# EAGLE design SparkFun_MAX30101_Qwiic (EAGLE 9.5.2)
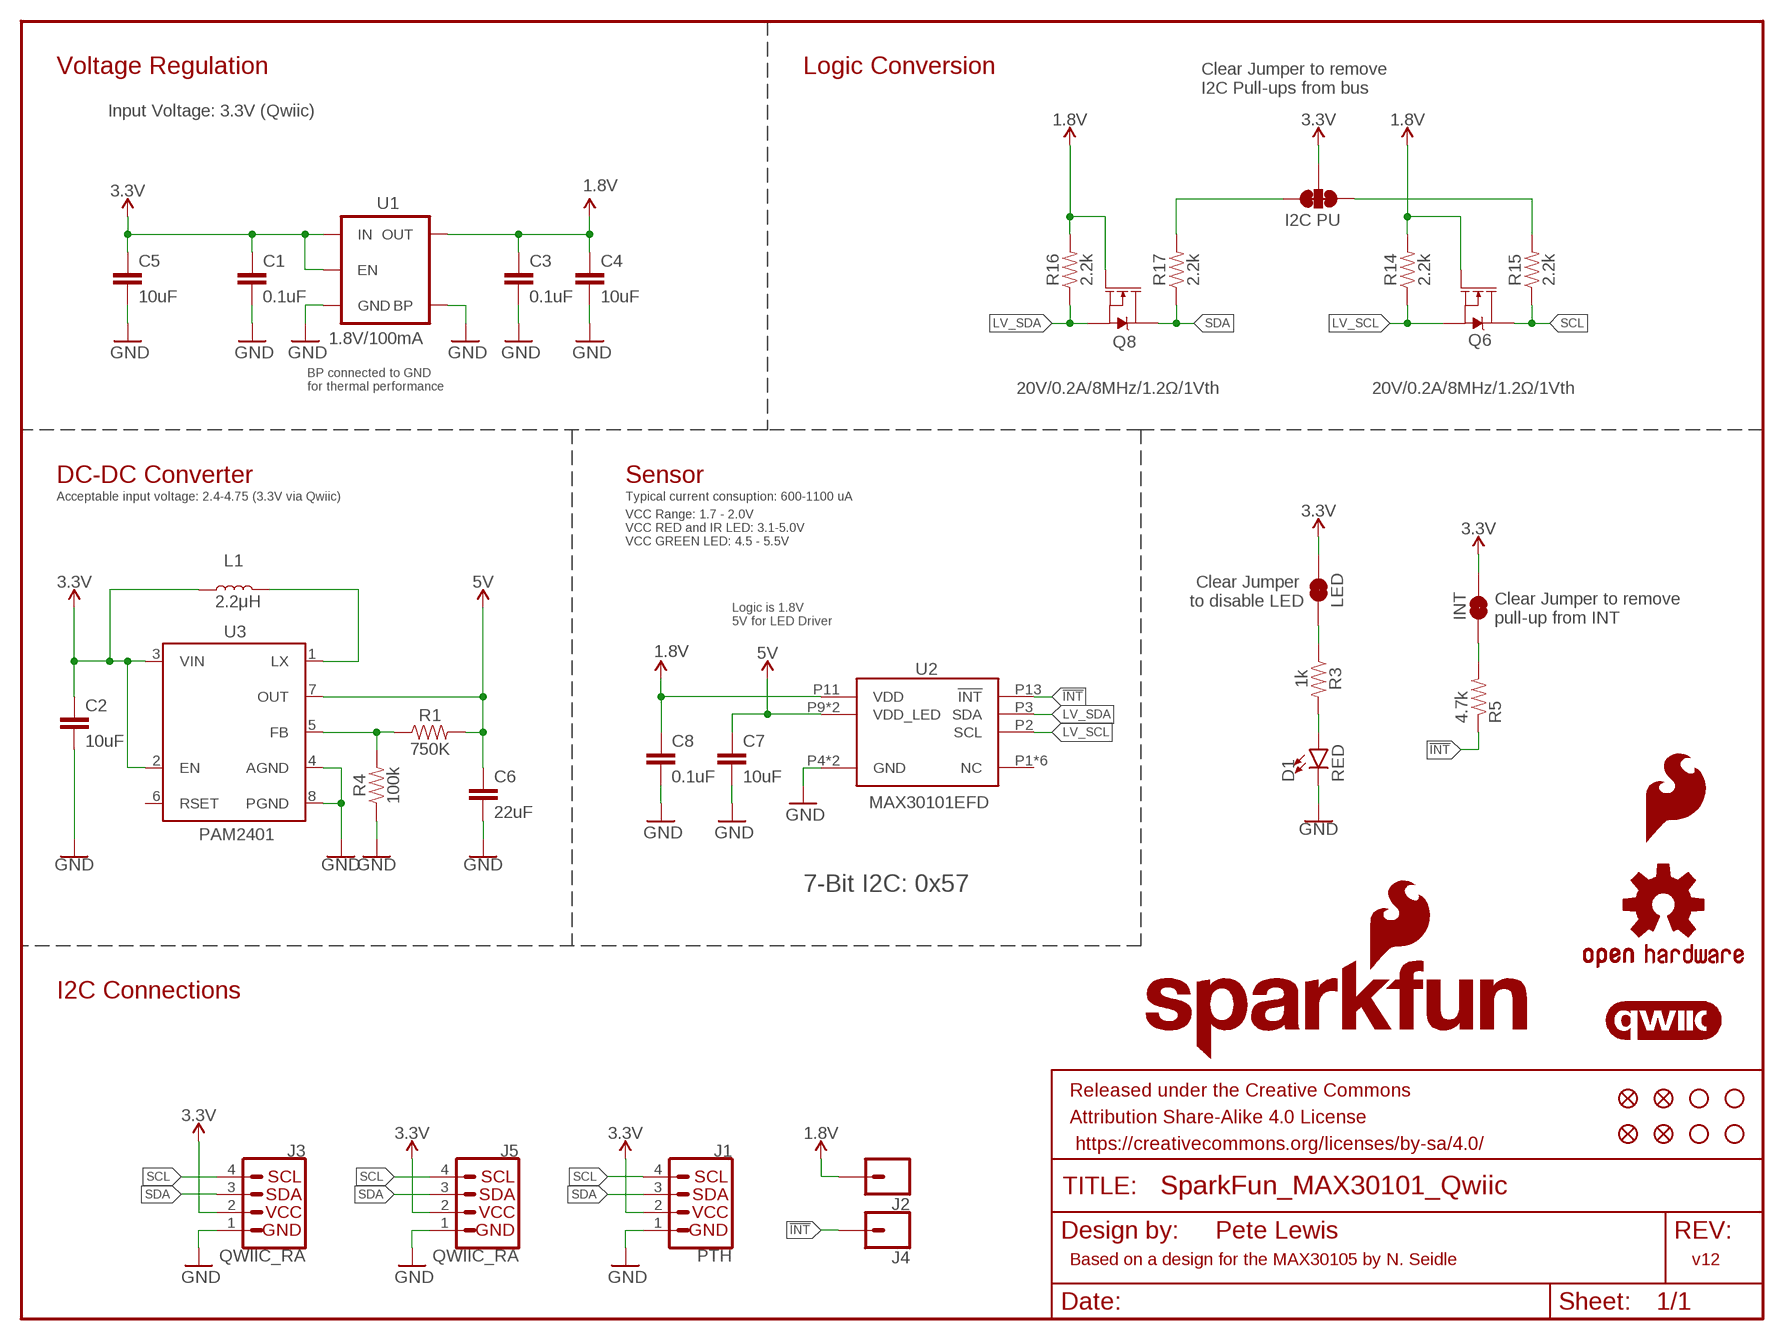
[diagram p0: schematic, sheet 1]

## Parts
C1  0.1uF  0.1UF-0402-16V-10%  [0402]
C2  10uF  10UF-0603-6.3V-20%  [0603]
C3  0.1uF  0.1UF-0402-16V-10%  [0402]
C4  10uF  10UF-0603-6.3V-20%  [0603]
C5  10uF  10UF-0603-6.3V-20%  [0603]
C6  22uF  22UF-0805-6.3V-20%  [0805]
C7  10uF  10UF-0603-6.3V-20%  [0603]
C8  0.1uF  0.1UF-0402-16V-10%  [0402]
D1  RED  LED-RED0603  [LED-0603]
FID1  FIDUCIAL1X2  [FIDUCIAL-1X2]
FID2  FIDUCIAL1X2  [FIDUCIAL-1X2]
FID3  FIDUCIAL1X2  [FIDUCIAL-1X2]
FID4  FIDUCIAL1X2  [FIDUCIAL-1X2]
FRAME1  FRAME-LETTER  [CREATIVE_COMMONS]
J1  PTH  I2C_STANDARD_NO_SILK  [1X04_NO_SILK]
J2  CONN_01PTH_NO_SILK_YES_STOP  [1X01_NO_SILK]
J3  QWIIC_RA  QWIIC_CONNECTORJS-1MM  [JST04_1MM_RA]
J4  CONN_01PTH_NO_SILK_YES_STOP  [1X01_NO_SILK]
J5  QWIIC_RA  QWIIC_CONNECTORJS-1MM  [JST04_1MM_RA]
JP1  LED  JUMPER-SMT_2_NC_TRACE_SILK  [SMT-JUMPER_2_NC_TRACE_SILK]
JP2  INT  JUMPER-SMT_2_NC_TRACE_SILK  [SMT-JUMPER_2_NC_TRACE_SILK]
JP4  I2C PU  JUMPER-SMT_3_2-NC_TRACE_SILK  [SMT-JUMPER_3_2-NC_TRACE_SILK]
L1  2.2μH  2.2μH_SHIELDED_INDUCTOR  [0806]
LOGO1  SFE_LOGO_NAME_FLAME.1_INCH  [SFE_LOGO_NAME_FLAME_.1]
LOGO2  OSHW-LOGOS  [OSHW-LOGO-S]
LOGO3  QWIIC_LOGO_5MM  [QWIIC_5MM]
LOGO4  SFE_LOGO_FLAME.1_INCH  [SFE_LOGO_FLAME_.1]
Q6  20V/0.2A/8MHz/1.2Ω/1Vth  MOSFET-NCH-RE1C00UNTL  [SOT-416FL]
Q8  20V/0.2A/8MHz/1.2Ω/1Vth  MOSFET-NCH-RE1C00UNTL  [SOT-416FL]
R1  750K  750KOHM-0603-1/10W-1%  [0603]
R3  1k  1KOHM-0603-1/10W-1%  [0603]
R4  100k  100KOHM-0603-1/10W-1%  [0603]
R5  4.7k  4.7KOHM-0603-1/10W-1%  [0603]
R14  2.2k  2.2KOHM-0603-1/10W-1%  [0603]
R15  2.2k  2.2KOHM-0603-1/10W-1%  [0603]
R16  2.2k  2.2KOHM-0603-1/10W-1%  [0603]
R17  2.2k  2.2KOHM-0603-1/10W-1%  [0603]
STANDOFF1  STAND-OFF  [STAND-OFF]
STANDOFF2  STAND-OFF  [STAND-OFF]
STANDOFF3  STAND-OFF  [STAND-OFF]
STANDOFF4  STAND-OFF  [STAND-OFF]
U1  1.8V/100mA  V_REG_SP62141.8V  [SC70]
U2  MAX30101EFD  [14_PIN_OESIP]
U3  PAM2401  [MSOP8]

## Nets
1.8V: C3.1 C4.1 C8.1 J2.1 Q6.1(G) Q8.1(G) R14.2 R16.2 U1.5(OUT) U2.P11(VDD)
3.3V: C1.1 C2.1 C5.1 J1.2 J3.2 J5.2 JP1.2 JP2.2 JP4.2 L1.1 U1.1(IN) U1.3(EN) U3.2(EN) U3.3(VIN)
5V: C6.1 C7.1 R1.2 U2.P9(VDD_LED) U2.P10(VDD_LED) U3.7(OUT)
!INT: J4.1 R5.1 U2.P13(!INT)
GND [power]: C1.2 C2.2 C3.2 C4.2 C5.2 C6.2 C7.2 C8.2 D1.C J1.1 J3.1 J5.1 R4.1 U1.2(GND) U1.4(BP) U2.P4(GND) U2.P12(GND) U3.4(AGND) U3.8(PGND)
LV_SCL: Q6.2(S) R14.1 U2.P2(SCL)
LV_SDA: Q8.2(S) R16.1 U2.P3(SDA)
N$1: JP2.1 R5.2
N$2: R1.1 R4.2 U3.5(FB)
N$3: L1.2 U3.1(LX)
N$4: D1.A R3.2
N$5: JP4.3 R15.2
N$6: JP4.1 R17.2
N$8: JP1.1 R3.1
SCL: J1.4 J3.4 J5.4 Q6.3(D) R15.1
SDA: J1.3 J3.3 J5.3 Q8.3(D) R17.1
Unconnected: U2.P1(NC) U2.P5(NC) U2.P6(NC) U2.P7(NC) U2.P8(NC) U2.P14(NC) U3.6(RSET)

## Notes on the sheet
- Voltage Regulation | Logic Conversion
- Clear Jumper to remove 
  I2C Pull-ups from bus
- Input Voltage: 3.3V (Qwiic)
- BP connected to GND
  for thermal performance
- DC-DC Converter | Sensor
- Acceptable input voltage: 2.4-4.75 (3.3V via Qwiic) | Typical current consuption: 600-1100 uA
- VCC Range: 1.7 - 2.0V
  VCC RED and IR LED: 3.1-5.0V
  VCC GREEN LED: 4.5 - 5.5V
- Clear Jumper 
  to disable LED
- Clear Jumper to remove 
  pull-up from INT
- Logic is 1.8V
  5V for LED Driver
- 7-Bit I2C: 0x57
- I2C Connections
- Pete Lewis
- Based on a design for the MAX30105 by N. Seidle | v12

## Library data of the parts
C1 C3 C8 = SparkFun-Capacitors:0.1UF: 0.1µF ceramic capacitors; PROD_ID: CAP-12416
C2 C4 C5 C7 = SparkFun-Capacitors:10UF: 10.0µF ceramic capacitors; PROD_ID: CAP-11015
C6 = SparkFun-Capacitors:22UF: 22µF ceramic capacitors; PROD_ID: CAP-08402
D1 = SparkFun-LED:LED-RED: Red SMD LED; PROD_ID: DIO-00819
FID1-FID4 = SparkFun-Aesthetics:FIDUCIAL: Fiducial Alignment Points
FRAME1 = SparkFun-Aesthetics:FRAME-LETTER: Schematic Frame - Letter
J1 = SparkFun-Connectors:I2C_STANDARD: SparkFun I2C Standard Pinout Header SparkFun has standardized on a pinout for all I2C based sensor breakouts. This pinout allows I2C boards to be plugged directly into the headers on Arduino Uno compatible boards, and to be daisy chained easily. Example SparkFun Products: SparkFun Atmospheric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
J2 J4 = SparkFun-Connectors:CONN_01: Single connection point. Often used as Generic Header-pin footprint for 0.1 inch spaced/style header connections
J3 J5 = SparkFun-Connectors:QWIIC_CONNECTOR: SparkFun I2C Standard Qwiic Connector An SMD 1mm pitch JST connector makes it easy and quick (get it? Qwiic?) to connect I2C devices to each other. The Qwiic system enables fast and solderless connection between popular platforms and various sensors and actuators. We carry 200mm, 100mm, 50mm, and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; PROD_ID: CONN-13694; VALUE: QWIIC_RIGHT_ANGLE
JP1 JP2 = SparkFun-Jumpers:JUMPER-SMT_2_NC_TRACE: Normally closed trace jumper
JP4 = SparkFun-Jumpers:JUMPER-SMT_3_2-NC_TRACE: Normally closed trace jumper (2 of 2 connections) This jumper has a trace between all three pads so they are normally closed (NC). Use a razor knife to open the connection(s). For best results follow the IPC guidelines for cutting traces: Cutout at least 0.063 mm (0.005 in). Remove all loose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
L1 = SparkFun-Coils:2.2μH_SHIELDED_INDUCTOR: Murata 2.2uH Inductor; PROD_ID: NDUC-14257
LOGO1 = SparkFun-Aesthetics:SFE_LOGO_NAME_FLAME: SparkFun Font Logo w/ Flame
LOGO2 = SparkFun-Aesthetics:OSHW-LOGO: Open-Source Hardware (OSHW) Logo
LOGO3 = SparkFun-Aesthetics:QWIIC_LOGO: Qwiic Logos for placement on schematic and PCB. The 5.5mm silk logo is best for placing next to Qwiic connector.
LOGO4 = SparkFun-Aesthetics:SFE_LOGO_FLAME: SparkFun Flame Logo
Q6 Q8 = SparkFun-DiscreteSemi:MOSFET-NCH: N-channel MOSFETs Voltage controlled devices that allow control of high current outputs. SparkFun Products: SparkFun OpenScale SparkFun Digital Sandbox SparkFun Monster Moto Shield SparkFun MOSFET Power Controller; PROD_ID: TRANS-14399
R1 = SparkFun-Resistors:750KOHM: 750Ω resistor; PROD_ID: RES-13768
R3 = SparkFun-Resistors:1KOHM: 1kΩ resistor; PROD_ID: RES-07856
R4 = SparkFun-Resistors:100KOHM: 100kΩ resistor; PROD_ID: RES-07828
R5 = SparkFun-Resistors:4.7KOHM: 4.7kΩ resistor; PROD_ID: RES-07857
R14-R17 = SparkFun-Resistors:2.2KOHM: 2.2kΩ resistor; PROD_ID: RES-08272
STANDOFF1-STANDOFF4 = SparkFun-Electromechanical:STAND-OFF: #4 Stand Off
U1 = SparkFun-PowerIC:V_REG_SP6214; PROD_ID: VREG-08428
U2 = SparkFun-IC-Special-Function:MAX30101EFD: MAX30101 High-Sensitivity Pulse Oximeter and Heart-Rate Sensor The MAX30101 is an integrated pulse oximetry and heart-rate monitor module. It includes internal LEDs, photodetectors, optical elements, and low-noise electronics with ambient light rejection. The MAX30101 provides a complete system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; PROD_ID: IC-14270
U3 = SparkFun-IC-Power:PAM2401: PAM2401 - Boost PMIC Specifications: Up to 1A output current 0.9V to 4.75V Input Range 2.5V to 5.0V Adjustable Output Voltage Datasheet (Diodes inc.); PROD_ID: IC-13769

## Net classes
1 power: width 0.203 mm

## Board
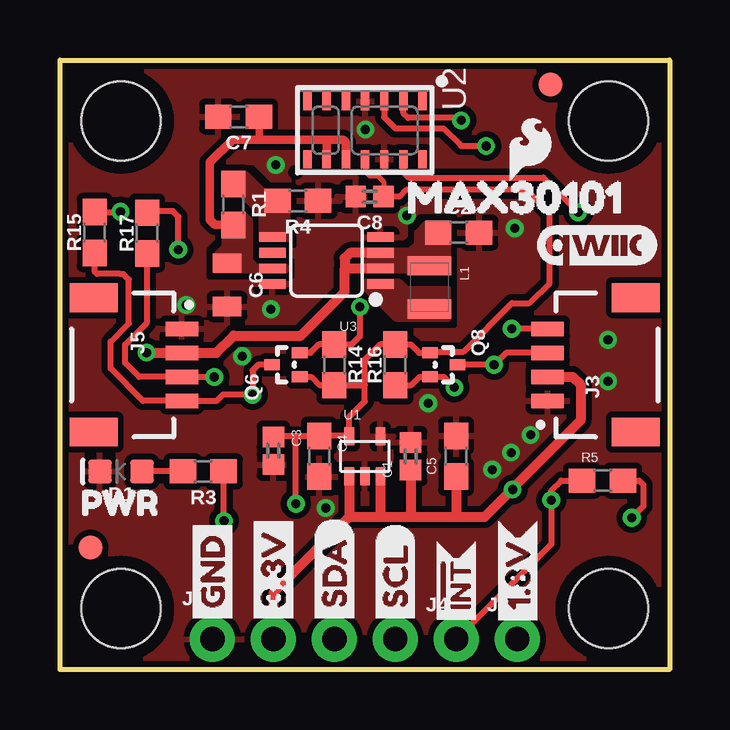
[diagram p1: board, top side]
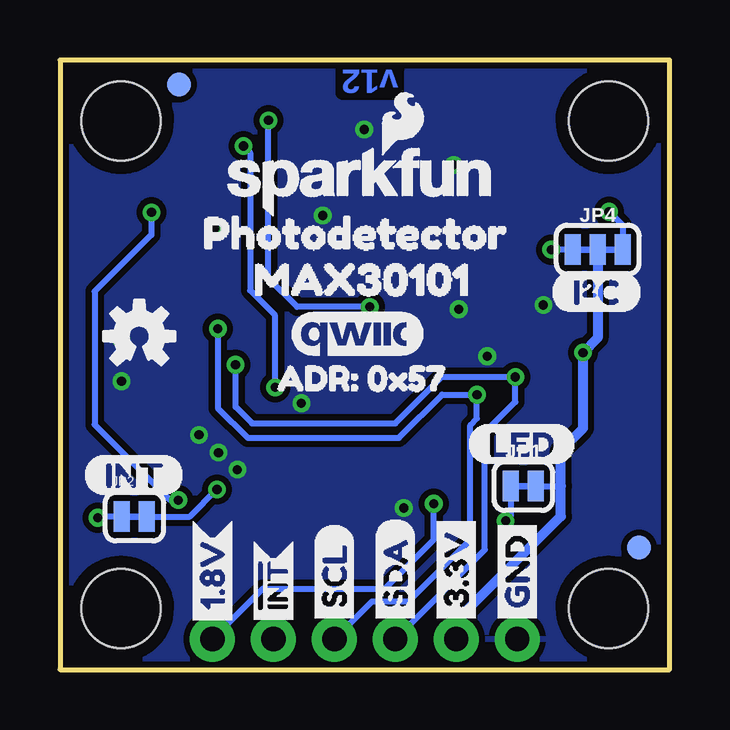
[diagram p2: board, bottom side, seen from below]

Size 25.4 x 25.4 mm. Coordinates in mm from the lower left corner, seen from the top.
Outline: 25.4,25.4 25.4,0 0,0 0,25.4 25.4,25.4
Copper layers (1*16): Top 0.035mm / dielectric 1.5mm / Bottom 0.035mm
Design rules "SparkFun-2-layer-TIGHT": minimum track width 7mil, minimum drill 15mil, track to track 7mil, track to pad 7mil, pad to pad 7mil, via to via 7mil, smd to smd 7mil, copper to edge 7mil, drill to drill 7mil, minimum pad ring 7mil, minimum via ring 7mil, stop-mask expansion 4mil, vias tented up to drill 25mil, thermal gap 10mil

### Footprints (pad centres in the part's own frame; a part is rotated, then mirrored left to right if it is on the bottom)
0402 = smd 0.85 x 0.9: 1 -0.58,0; 2 0.58,0
0603 = smd 1.1 x 1: 1 -0.85,0; 2 0.85,0
0805 = smd 0.8 x 1.2: 1 -0.9,0; 2 0.9,0
LED-0603 = smd 1 x 1: A -0.877,0; C 0.877,0
FIDUCIAL-1X2 = smd 1 x 1: 1 0,0
1X04_NO_SILK = drill 1.016 pad 1.88: 1 0,0; 2 2.54,0; 3 5.08,0; 4 7.62,0
1X01_NO_SILK = drill 1.016 pad 1.88: 1 0,0
JST04_1MM_RA = smd 0.6 x 1.35: 1 -1.5,0; 2 -0.5,0; 3 0.5,0; 4 1.5,0 | smd 1.2 x 2: NC1 2.8,-3.675; NC2 -2.8,-3.675
SMT-JUMPER_2_NC_TRACE_SILK = smd 0.66 x 1.27: 1 -0.521,0; 2 0.521,0
SMT-JUMPER_3_2-NC_TRACE_SILK = smd 0.66 x 1.27: 1 -1.041,0; 2 0,0; 3 1.041,0
0806 = smd 0.8 x 1.8: 1 -0.9,0; 2 0.9,0
SOT-416FL = smd 0.46 x 0.65: 1 -0.5,-1.1; 2 0.5,-1.1; 3 0,0.05
STAND-OFF = hole 3.302: 0,0
SC70 = smd 0.4 x 0.75: 1 -0.65,-0.825; 2 0,-0.825; 3 0.65,-0.825; 4 0.65,0.825; 5 -0.65,0.825
14_PIN_OESIP = smd 0.75 x 0.35: P1 -1.193,2.409; P2 -1.193,1.609; P3 -1.193,0.809; P4 -1.193,0.009; P5 -1.193,-0.791; P6 -1.193,-1.591; P7 -1.193,-2.391; P8 1.207,-2.391; P9 1.207,-1.591; P10 1.207,-0.791; P11 1.207,0.009; P12 1.207,0.809; P13 1.207,1.609; P14 1.207,2.409
MSOP8 = smd 0.4 x 1.1: 1 -0.975,-2.25; 2 -0.325,-2.25; 3 0.325,-2.25; 4 0.975,-2.25; 5 0.975,2.25; 6 0.325,2.25; 7 -0.325,2.25; 8 -0.975,2.25

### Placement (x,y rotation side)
C1  14.61,8.89 90 top
C2  16.61,18.21 0 top
C3  8.89,9.12 270 top
C4  10.79,8.89 270 top
C5  16.51,8.89 90 top
C6  6.96,16.03 270 top
C7  7.44,23.04 180 top
C8  12.9,19.71 180 top
D1  2.54,8.26 180 top
FID1  20.45,24.38 90 top
FID2  1.27,5.08 90 top
FID3  20.45,24.38 0 bottom
FID4  1.27,5.08 0 bottom
FRAME1  not placed on the board
J1  6.35,1.27 0 top
J2  19.05,1.27 0 top
J3  20.32,12.7 90 top
J4  16.51,1.27 0 top
J5  5.08,12.7 270 top
JP1  6.1,7.65 0 bottom
JP2  22.3,6.38 0 bottom
JP4  3,17.5 0 bottom
L1  15.39,15.93 270 top
LOGO1  12.85,20.35 0 bottom
LOGO2  22.1,13.89 0 bottom
LOGO3  22.35,17.7 0 top
LOGO4  19.58,21.69 0 top
Q6  8.89,12.7 90 top
Q8  16.51,12.7 270 top
R1  7.21,19.38 270 top
R3  5.97,8.26 180 top
R4  9.91,19.53 180 top
R5  22.61,7.87 0 top
R14  11.43,12.7 270 top
R15  1.45,18.21 90 top
R16  13.97,12.7 90 top
R17  3.63,18.19 90 top
STANDOFF1  2.54,22.86 90 top
STANDOFF2  22.86,22.86 90 top
STANDOFF3  22.86,2.54 90 top
STANDOFF4  2.54,2.54 90 top
U1  12.7,8.89 0 top
U2  12.7,22.48 270 top
U3  11.1,17.04 90 top
U$1  [PHOTODETECTOR3]  20.6,18.19 0 bottom
U$3  [INT#-[<-04]  16.51,1.4 90 top
U$4  [MAX301010]  13.31,19.68 0 top
U$7  [INT-()-04]  24.46,8.1 0 bottom
U$8  [LED0]  8.46,9.4 0 bottom
U$9  [SCL-[)]  13.97,1.65 90 bottom
U$10  [GND-04]  6.35,1.65 90 top
U$11  [INT#-[<-04]  16.51,1.4 90 bottom
U$12  [SCL-[)]  13.97,1.65 90 top
U$13  [SDA-[)]  11.43,1.65 90 top
U$14  [SDA-[)]  11.43,1.65 90 bottom
U$15  [ADR#_0X570]  17.22,12.14 0 bottom
U$16  [QWIIC_5.5MM]  13,14 0 bottom
U$19  [3.3V]  8.89,1.65 90 top
U$20  [1#8V0]  19.08,1.57 90 top
U$21  [I_SUPER2_C-()-04]  4.95,15.72 0 bottom
U$22  [3.3V]  8.89,1.65 90 bottom
U$23  [GND-04]  6.35,1.65 90 bottom
U$24  [MAX301010]  18.47,16.26 0 bottom
U$26  [PWR_TO]  -0.03,6.96 0 top
U$27  [1#8V0]  19.05,1.57 90 bottom

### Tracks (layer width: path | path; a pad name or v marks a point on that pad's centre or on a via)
1.8V  (via drill 0.38)
  Top 0.203: U2.P11 12.71,20.77 12.9,20.57 13.23,20.57 13.48,20.32 C8.1
  Top 0.254: 12.7,11.86 12.7,11.18 12.05,10.53 U1.5 12.03,9.74 C4.1 9.83,9.74 | 12.7,11.86 12.7,12.9 13.35,13.55 R16.2 14.62,13.55 14.97,13.2 Q8.1 15.46,13.25 16.82,13.25 18.83,15.27 19.56,15.27 20.4,16.1 20.4,19.02 19.43,19.99 14.43,19.99 14.15,19.71 C8.1 | 12.7,11.86 12.69,11.85 R14.2 10.83,11.85 10.48,12.2 Q6.1 | v9.83,6.91 9.83,9.74 | C3.1 8.93,9.74 9.83,9.74
  Bottom 0.254: J2.1 16.94,3.38 11.86,3.38 9.83,5.41 v9.83,6.91
3.3V  (via drill 0.38)
  Top 0.406: J3.2 21.35,12.2 21.69,11.86 21.69,10.39 18.86,7.56 v18.86,7.51 18.83,7.51 17.68,6.35 16.51,6.35 | 16.51,6.35 14.61,6.35 | 14.61,6.35 13.34,6.35 | U1.3 13.35,6.37 13.34,6.35 | C1.1 14.61,6.35 | C5.1 16.51,6.35 | J1.2 8.89,3.2 12.04,6.35 | 13.34,6.35 12.04,6.35 | U1.1 12.05,6.36 12.04,6.35 | v3.61,13.21 J5.2 6.52,13.2 7.24,13.92 10.03,13.92 11.86,15.75 11.86,16.66 | 11.86,16.66 11.92,16.72 U3.2 | U3.3 12.09,17.37 11.86,17.14 11.86,16.66
  Bottom 0.254: JP2.2 19.99,6.38 v18.86,7.51 | JP1.2 4.53,7.64
  Bottom 0.406: J1.2 8.89,2.03 4.53,6.39 4.53,7.64 4.53,9.13 3.61,10.06 v3.61,13.21 3,13.82 JP4.2
  pour Top (no thermals): 16.21,18.62 15.24,18.62 14.83,18.21 14.83,17.73 14.58,17.48 12.78,17.48 12.78,16.61 14.45,16.61 14.53,16.54 16.21,16.54
5V
  Top 0.305: C7.1 8.29,22.08 8.28,22.07
  Top 0.356: 11.1,22.07 11.81,22.07 11.91,21.98 U2.P10 | 11.1,22.07 8.28,22.07 7.19,22.07 6.25,21.13 6.25,18.75 6.45,18.54 7.2,18.54 R1.2 | U2.P9 11.11,22.06 11.1,22.07
  pour Top (no thermals): 9.42,16.81 8.18,16.81 7.95,17.04 7.95,18.69 7.67,18.97 6.83,18.97 6.83,17.63 6.45,17.25 6.45,16.61 9.42,16.61
!INT  (via drill 0.38)
  Top 0.254: v21.59,19.05 20.14,20.5 14.53,20.5 14.32,20.7 14.31,20.72 U2.P13 | R5.1 20.88,7.87 20.47,7.47 v20.47,7.06 20.47,5.23 J4.1
  Bottom 0.254: v21.59,19.05 21.59,18.12 23.95,15.75 23.95,10.21 20.8,7.06 v20.47,7.06
GND  (via drill 0.38)
  other vias: 11.07,6.73 15.34,11.1 18.01,8.33 19.61,9.78 5.26,15.19 12.73,22.5 7.59,13.06 18.8,9.04 22.83,13.74 22.83,12.01 14.45,18.92 18.95,18.39 8.79,15.01 8.99,21.03
  pour Top (isolate 0.254, rank 6): 0,25.4 0,0 25.4,0 25.4,25.4
  pour Bottom (isolate 0.254, rank 6): 0,25.4 0,0 25.4,0 25.4,25.4
LV_SCL  (via drill 0.38)
  Top 0.254: Q6.2 10.43,13.2 10.78,13.55 R14.1 12.17,13.55 12.5,13.88 v12.5,15.11 | v16.71,22.89 16.61,22.99 14.5,22.99 14.31,23.18 U2.P2
  Bottom 0.254: v12.5,15.11 15.52,15.11 16.71,16.31 v16.71,22.89
LV_SDA  (via drill 0.38)
  Top 0.254: R16.1 14.64,11.85 14.99,12.2 Q8.2 15.99,12.2 v16.43,11.76 | v17.75,21.82 16.71,21.82 15.98,22.55 13.97,22.55 13.51,23.02 U2.P3
  Bottom 0.254: v16.43,11.76 16.43,14.76 17.48,15.8 17.48,21.54 v17.75,21.82
N$1  (via drill 0.38)
  Top 0.254: R5.2 24.13,7.87 24.31,7.7 24.31,6.81 v23.82,6.33
  Bottom 0.254: JP2.1 23.77,6.38 v23.82,6.33
N$2
  pour Top (no thermals): 8.38,17.91 8.38,18.95 7.54,19.79 6.83,19.79 6.83,20.68 7.75,20.68 8.51,19.91 9.5,19.91 9.5,17.91
N$3
  pour Top (no thermals): 16.21,14.61 16.21,15.88 15.88,15.88 14.45,15.88 14.15,16.18 12.73,16.18 12.73,15.88 14,14.61
N$4
  Top 0.254: R3.2 D1.A
N$5  (via drill 0.38)
  Top 0.254: R15.2 2.51,19.06 v2.52,19.07
  Bottom 0.254: v2.52,19.07 1.96,18.51 JP4.3
N$6  (via drill 0.38)
  Top 0.254: v4.93,17.5 4.93,18.87 4.7,19.1 3.7,19.1 R17.2
  Bottom 0.254: JP4.1 v4.93,17.5
N$8  (via drill 0.38)
  Top 0.254: v6.83,6.2 6.82,6.21 R3.1
  Bottom 0.254: JP1.1 6.62,6.41 v6.83,6.2
SCL  (via drill 0.38)
  Top 0.254: R15.1 1.45,16.59 1.55,16.48 2.51,16.48 2.64,16.48 2.87,16.25 2.87,14.43 2.11,13.66 2.11,12.55 3.46,11.2 J5.4 6.53,11.2 6.78,11.46 v8.03,11.46 8.03,12.47 8.26,12.7 Q6.3 | J3.4 v18.82,14.2
  Bottom 0.254: v18.82,14.2 18.82,10.9 17.58,9.65 11.28,9.65 9.47,11.46 v8.03,11.46 8.03,10.46 8.31,10.19 8.31,5.41 10.87,2.85 12.39,2.85 J1.4
SDA  (via drill 0.38)
  Top 0.254: R17.1 3.61,17.31 3.61,14.43 2.72,13.54 2.72,12.78 3.29,12.2 J5.3 6.42,12.2 v6.43,12.19 | J3.3 18.59,13.2 v18.09,12.7 Q8.3
  Bottom 0.254: v18.09,12.7 18.09,10.95 17.4,10.26 11.43,10.26 9.5,12.19 v6.43,12.19 6.43,11.15 7.7,9.88 7.7,5 J1.3

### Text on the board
Bottom: v12
tDocu: Pete Lewis | Based on a design for the MAX30105 by N. Seidle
